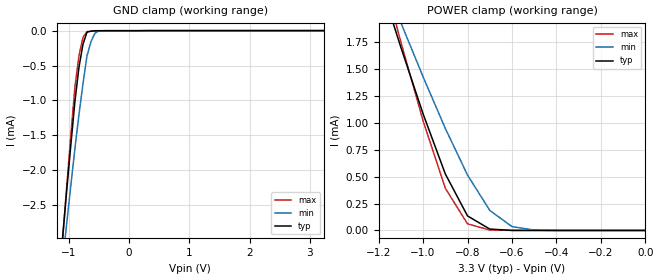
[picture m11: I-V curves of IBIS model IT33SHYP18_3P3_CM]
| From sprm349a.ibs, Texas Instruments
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|   Model Cell IT33SHYP18_3P3_CM
|IT33SHYP18_3P3
[Model]   IT33SHYP18_3P3_CM
Model_type   Input
Polarity   Non-Inverting
Vinl =  0.8V
Vinh =  2V
C_comp   0.7465841p   0.68548p   0.8226742p
[Model Spec]
Vinl   0.8V   0.8V   0.8V
Vinh   2V   2V   2V
[Temperature Range]   25   105   0
[Voltage Range]   3.3   2.97   3.63
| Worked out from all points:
|   GND clamp passes 1 mA (typ) near -0.90 V on its own axis
|   POWER clamp passes 1 mA (typ) near -0.98 V on its own axis
[POWER_clamp]
|   voltage   I(typ)   I(min)   I(max)
-3.3V     16.09mA    13.57mA    18.61mA
-1.133V   1.92mA     2.105mA    2.012mA
-1.1V     1.705mA    1.933mA    1.754mA
-1.067V   1.498mA    1.765mA    1.51mA
-1V       1.085mA    1.429mA    1.021mA
-900mV    526.2uA    949uA      393.3uA
-800mV    135.4uA    515.1uA    61.69uA
-700mV    13.19uA    186.7uA    3.903uA
-600mV    617.4nA    36.16uA    891.7nA
-500mV    119.1nA    3.777uA    813.5nA
-11.55fV  95.16nA    41.34nA    731.3nA
[GND_clamp]
|   voltage   I(typ)   I(min)   I(max)
-3.3V     -25.77mA   -21.96mA   -28.61mA
-1.1V     -2.914mA   -3.271mA   -2.94mA
-1.033V   -2.256mA   -2.732mA   -2.191mA
-966.7mV  -1.62mA    -2.203mA   -1.477mA
-900mV    -1.008mA   -1.684mA   -799.5uA
-833.3mV  -523.5uA   -1.201mA   -356.6uA
-766.7mV  -194.5uA   -760.2uA   -94.57uA
-700mV    -20.9uA    -361.1uA   -13.52uA
-633.3mV  -8.234uA   -155.2uA   -6.943uA
-566.7mV  -1.665uA   -35.94uA   -3.506uA
-500mV    -1.19uA    -3.305uA   -3.211uA
3.233V    93.9nA     54.41nA    675.9nA
